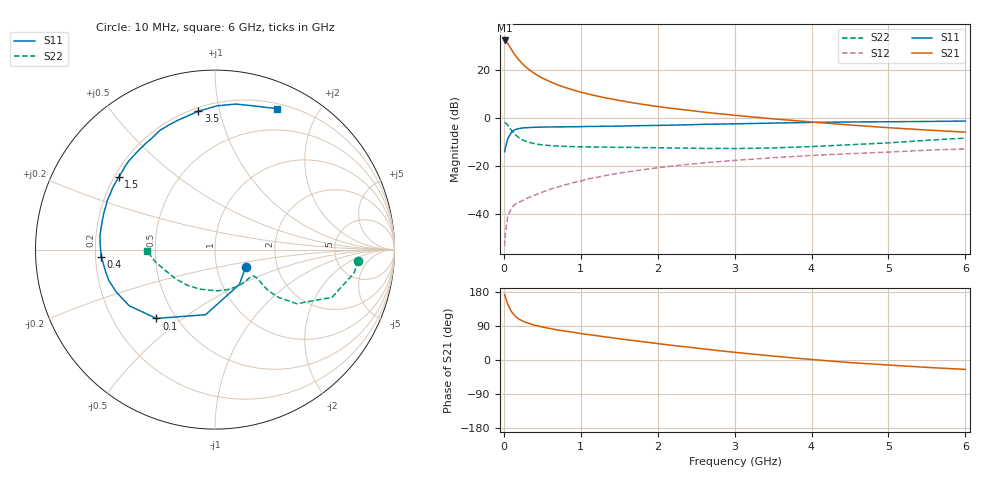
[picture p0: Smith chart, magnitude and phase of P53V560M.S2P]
! SIEMENS Small Signal Semiconductors
! BFP183
! Si NPN RF Bipolar Junction Transistor in SOT143
! VCE = 3.5 V  IC = 60 mA
! Common Emitter S-Parameters:  March  1996
# GHz  S  MA  R  50
!  f  S11  S21  S12  S22
! GHz  MAG  ANG  MAG  ANG  MAG  ANG  MAG  ANG
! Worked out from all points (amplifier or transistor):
!   36 points, 10 MHz to 6 GHz, reference 50 ohm
!   highest |S21| = 32.3 dB at 10 MHz (marker M1)
!   |S21| within 3 dB of that: start of sweep to 83.62 MHz
!   unconditionally stable (mu >= 1): start of sweep to 25.06 MHz; 239 MHz to end of sweep
!   at 250 MHz: K = 1.02, MAG = 27.4 dB, |S12| = -34.4 dB
!   at 1.4 GHz: K = 1.53, MAG = 11.5 dB, |S12| = -23.6 dB
!   at 6 GHz: K = 1.15, MAG = 1.2 dB, |S12| = -13.0 dB
!   S11 on the Smith chart (normalised r, x): 10 MHz: 1.38, -0.28; 100 MHz: 0.39, -0.40; 400 MHz: 0.22, -0.03; 1.5 GHz: 0.22, +0.32; 3.5 GHz: 0.22, +0.86; 6 GHz: 0.25, +1.50
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0.01  0.1975 -30.2  41.1 172.9  0.0021 65.4  0.8002 -4.4
0.02  0.2368 -55.0  40.41 166.3  0.0038 69.1  0.7861 -9.5
0.05  0.3663 -98.2  35.79 147.7  0.0088 65.5  0.704 -22.2
0.1  0.5037 -130.4  26.31 127.3  0.013 51.2  0.5463 -33.5
0.15  0.5719 -146.9  19.96 115.2  0.016 48.7  0.4442 -36.9
0.2  0.5991 -156.9  15.8 107.5  0.0173 49.1  0.3807 -37.6
0.25  0.6159 -163.7  12.99 102.2  0.019 49.3  0.3431 -36.9
0.3  0.622 -168.9  11 98.2  0.0209 51.9  0.3175 -35.8
0.4  0.6348 -176.5  8.382 91.8  0.0242 55.5  0.2881 -34.5
0.5  0.6404 177.4  6.735 87.1  0.0281 56.9  0.2722 -34.1
0.6  0.6455 173.0  5.686 83.0  0.0322 59.0  0.2635 -34.3
0.7  0.6463 168.8  4.853 79.4  0.036 60.9  0.2573 -34.9
0.9  0.6521 161.7  3.82 73.2  0.0444 61.9  0.251 -37.5
1.1  0.6605 154.9  3.131 67.0  0.0532 61.6  0.2462 -41.0
1.5  0.6711 143.0  2.304 56.0  0.0703 60.0  0.2426 -49.3
1.8  0.6882 134.6  1.918 48.3  0.0824 57.9  0.2385 -57.0
2.2  0.7039 124.4  1.564 38.4  0.0991 54.2  0.2342 -67.8
2.8  0.7401 110.3  1.218 24.5  0.1219 48.1  0.2301 -86.6
3.5  0.7766 96.8  0.952 10.3  0.147 41.5  0.2356 -110.5
4.5  0.819 81.9  0.708 -6.9  0.1787 31.4  0.2742 -144.0
5.5  0.8392 71.0  0.556 -19.5  0.2115 22.3  0.3398 -168.5
6  0.8571 66.4  0.502 -24.8  0.2243 17.2  0.3777 -178.8
